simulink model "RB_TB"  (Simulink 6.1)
settings: Solver=ode3  SolverMode=SingleTasking  StartTime=0  StopTime=0.1  FixedStep=0.01  RelTol=1e-3
libraries: simulink x2
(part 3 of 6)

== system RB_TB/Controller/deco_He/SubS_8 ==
  note: Model: RB_TB/Controller/deco_He/SubS_2
  Palv : Inport  Port=1  LatchInput=off
  Pamb_sea : Inport  Port=2  LatchInput=off
  Palv_INI : Inport  Port=3  LatchInput=off
  HT : Inport  Port=4  LatchInput=off
  BC1 : BusCreator  DialogController=Simulink.DDGSource_Bus
  He_a : Constant  Value=0.6508
  He_b : Constant  Value=0.8553
  Mux6 : Mux  Inputs=3
  Product1 : Product
  Sum2 : Sum  Inputs=|+-
  Sum3 : Sum  Inputs=++|
  fcn1 : Fcn  Expr=log(2)/u(1)
  fcn3 : Fcn  Expr=u(3)+u(2)/u(1)
  pr_PHe : TransferFcn  Numerator=[1/60]  Denominator=[1 0]
  bus : Outport
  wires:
  HT/1 -> fcn1/1
  Sum2/1 -> Product1/2
  Product1/1 -> pr_PHe/1
  fcn3/1 -> BC1/4  "M0"
  He_b/1 -> BC1/3, Mux6/1  "He_b"
  Mux6/1 -> fcn3/1
  fcn1/1 -> BC1/1, Product1/1  "He_k"
  Palv/1 -> Sum2/1
  Pamb_sea/1 -> Mux6/2
  He_a/1 -> Mux6/3  "He_a"
  Sum3/1 -> Sum2/2, BC1/2  "Pt"
  Palv_INI/1 -> Sum3/1
  pr_PHe/1 -> Sum3/2
  BC1/1 -> bus/1

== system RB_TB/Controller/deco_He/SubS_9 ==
  note: Model: RB_TB/Controller/deco_He/SubS_2
  Palv : Inport  Port=1  LatchInput=off
  Pamb_sea : Inport  Port=2  LatchInput=off
  Palv_INI : Inport  Port=3  LatchInput=off
  HT : Inport  Port=4  LatchInput=off
  BC1 : BusCreator  DialogController=Simulink.DDGSource_Bus
  He_a : Constant  Value=0.5981
  He_b : Constant  Value=0.8757
  Mux6 : Mux  Inputs=3
  Product1 : Product
  Sum2 : Sum  Inputs=|+-
  Sum3 : Sum  Inputs=++|
  fcn1 : Fcn  Expr=log(2)/u(1)
  fcn3 : Fcn  Expr=u(3)+u(2)/u(1)
  pr_PHe : TransferFcn  Numerator=[1/60]  Denominator=[1 0]
  bus : Outport
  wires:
  BC1/1 -> bus/1
  pr_PHe/1 -> Sum3/2
  Palv_INI/1 -> Sum3/1
  Sum3/1 -> BC1/2, Sum2/2  "Pt"
  He_a/1 -> Mux6/3  "He_a"
  Pamb_sea/1 -> Mux6/2
  Palv/1 -> Sum2/1
  fcn1/1 -> Product1/1, BC1/1  "He_k"
  Mux6/1 -> fcn3/1
  He_b/1 -> Mux6/1, BC1/3  "He_b"
  fcn3/1 -> BC1/4  "M0"
  Product1/1 -> pr_PHe/1
  Sum2/1 -> Product1/2
  HT/1 -> fcn1/1

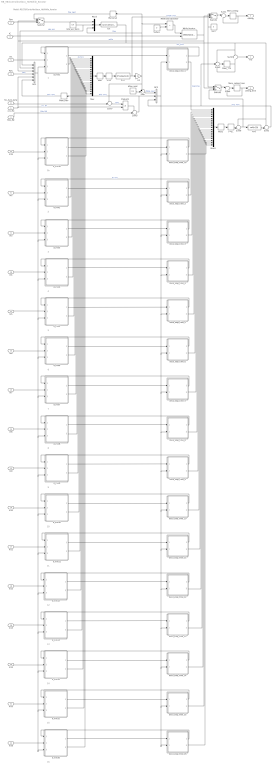
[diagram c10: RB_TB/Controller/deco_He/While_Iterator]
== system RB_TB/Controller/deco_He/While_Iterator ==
  note: 16
  note: 15
  note: 14
  note: 13
  note: 12
  note: 11
  note: 10
  note: 9
  note: 8
  note: 7
  note: 6
  note: 5
  note: 4
  note: 3
  note: 2
  note: 1
  note: Model: RB_TB/Controller/deco_He/While_Iterator
  note: 1b
  cnc_He : Inport  Port=1  LatchInput=off
  Psw : Inport  Port=2  LatchInput=off
  IC : Inport  Port=3  LatchInput=off
  Palv : Inport  Port=4  LatchInput=off
  In1 : Inport  Port=5  LatchInput=off
  In2 : Inport  Port=6  LatchInput=off
  Palv_INI : Inport  Port=7  LatchInput=off
  fnc_hum_temp : Inport  Port=8  LatchInput=off
  In3 : Inport  Port=9  LatchInput=off
  In4 : Inport  Port=10  LatchInput=off
  In5 : Inport  Port=11  LatchInput=off
  In6 : Inport  Port=12  LatchInput=off
  In7 : Inport  Port=13  LatchInput=off
  In8 : Inport  Port=14  LatchInput=off
  In9 : Inport  Port=15  LatchInput=off
  In10 : Inport  Port=16  LatchInput=off
  In11 : Inport  Port=17  LatchInput=off
  In12 : Inport  Port=18  LatchInput=off
  In13 : Inport  Port=19  LatchInput=off
  In14 : Inport  Port=20  LatchInput=off
  In15 : Inport  Port=21  LatchInput=off
  In16 : Inport  Port=22  LatchInput=off
  In1b : Inport  Port=23  LatchInput=off
  >=0 : DeadZone  LowerValue=-1000  UpperValue=0
  >=0_ : DeadZone  LowerValue=-inf  UpperValue=0
  BC1 : BusCreator  DialogController=Simulink.DDGSource_Bus  Inputs=6
  BC2 : BusCreator  DialogController=Simulink.DDGSource_Bus  Inputs=3
  K1 : Gain  Gain=0.1
  Max : MinMax  Function=max
  Max1 : MinMax  Function=max
  Mem_Palv : Memory  Orientation=left  InheritSampleTime=on
  Mem_TTS : Memory  InheritSampleTime=on
  Mem_ceiling : Memory  InheritSampleTime=on
  Mem_ceiling_time : Memory  InheritSampleTime=on
  Memory2 : Memory  Orientation=left  InheritSampleTime=on
  Mux : Mux  Inputs=17
  Mux1 : Mux  Inputs=17
  Mux3 : Mux  Inputs=3
  Product1 : Product
  Relational Operator : RelationalOperator  Operator=>  LogicOutDataTypeMode=Boolean
  Suface : Constant  Value=0
  Sum : Sum  Inputs=+-|
  Sum1 : Sum  Inputs=|++
  Sum2 : Sum  Inputs=-+|
  Sum3 : Sum  Inputs=+++
  Sum4 : Sum  Inputs=|++
  Sum5 : Sum
  Sum6 : Sum  Inputs=++|
  Sum7 : Sum  Inputs=++|
  Sum8 : Sum
  Switch1 : Switch  Threshold=2
  Switch2 : Switch  Threshold=2
  Switch3 : Switch  Threshold=2
  While Iterator : WhileIterator  MaxIters=100  ShowIterationPort=on
  dPsw_next : Constant  Value=0.3
  d_min1 : Subsystem
  d_min10 : Subsystem
  d_min11 : Subsystem
  d_min12 : Subsystem
  d_min13 : Subsystem
  d_min14 : Subsystem
  d_min15 : Subsystem
  d_min16 : Subsystem
  d_min1b : Subsystem
  d_min2 : Subsystem
  d_min3 : Subsystem
  d_min4 : Subsystem
  d_min5 : Subsystem
  d_min6 : Subsystem
  d_min7 : Subsystem
  d_min8 : Subsystem
  d_min9 : Subsystem
  deco_stop_time_1 : Subsystem
  deco_stop_time_10 : Subsystem
  deco_stop_time_11 : Subsystem
  deco_stop_time_12 : Subsystem
  deco_stop_time_13 : Subsystem
  deco_stop_time_14 : Subsystem
  deco_stop_time_15 : Subsystem
  deco_stop_time_16 : Subsystem
  deco_stop_time_1b : Subsystem
  deco_stop_time_2 : Subsystem
  deco_stop_time_3 : Subsystem
  deco_stop_time_4 : Subsystem
  deco_stop_time_5 : Subsystem
  deco_stop_time_6 : Subsystem
  deco_stop_time_7 : Subsystem
  deco_stop_time_8 : Subsystem
  deco_stop_time_9 : Subsystem
  fcn : Fcn  Expr=(u(1)-u(3))/u(2)
  fcn1 : Fcn  Expr=ceil(u(1))
  fcn2 : Fcn  Expr=3*ceil(u(1)/3)
  rate_asc_deco : Constant  Value=0.9
  zero : Constant  Orientation=left  Value=0
  TTS : Outport
  ceiling : Outport  Port=2
  ceiling_time : Outport  Port=3
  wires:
  deco_stop_time_16/2(deco_stop_time) -> Mux1/16
  deco_stop_time_15/2(deco_stop_time) -> Mux1/15
  deco_stop_time_14/2(deco_stop_time) -> Mux1/14
  deco_stop_time_13/2(deco_stop_time) -> Mux1/13
  deco_stop_time_12/2(deco_stop_time) -> Mux1/12
  deco_stop_time_11/2(deco_stop_time) -> Mux1/11
  deco_stop_time_10/2(deco_stop_time) -> Mux1/10
  deco_stop_time_9/2(deco_stop_time) -> Mux1/9
  deco_stop_time_8/2(deco_stop_time) -> Mux1/8
  deco_stop_time_7/2(deco_stop_time) -> Mux1/7
  deco_stop_time_6/2(deco_stop_time) -> Mux1/6
  deco_stop_time_5/2(deco_stop_time) -> Mux1/5
  deco_stop_time_4/2(deco_stop_time) -> Mux1/4
  deco_stop_time_3/2(deco_stop_time) -> Mux1/3
  d_min16/2(d_min) -> Mux/16
  d_min15/2(d_min) -> Mux/15
  d_min14/2(d_min) -> Mux/14
  d_min13/2(d_min) -> Mux/13
  d_min12/2(d_min) -> Mux/12
  d_min11/2(d_min) -> Mux/11
  d_min10/2(d_min) -> Mux/10
  d_min9/2(d_min) -> Mux/9
  d_min8/2(d_min) -> Mux/8
  d_min7/2(d_min) -> Mux/7
  d_min6/2(d_min) -> Mux/6
  d_min5/2(d_min) -> Mux/5
  d_min4/2(d_min) -> Mux/4
  d_min3/2(d_min) -> Mux/3
  deco_stop_time_2/2(deco_stop_time) -> Mux1/2
  Mux1/1 -> Max1/1
  d_min16/1(bus1) -> deco_stop_time_16/1(In1)
  deco_stop_time_16/1(Pt_new) -> d_min16/1(Pt_new)
  In16/1 -> d_min16/2(In1)
  In15/1 -> d_min15/2(In1)
  deco_stop_time_15/1(Pt_new) -> d_min15/1(Pt_new)
  d_min15/1(bus1) -> deco_stop_time_15/1(In1)
  d_min14/1(bus1) -> deco_stop_time_14/1(In1)
  deco_stop_time_14/1(Pt_new) -> d_min14/1(Pt_new)
  In14/1 -> d_min14/2(In1)
  In13/1 -> d_min13/2(In1)
  deco_stop_time_13/1(Pt_new) -> d_min13/1(Pt_new)
  d_min13/1(bus1) -> deco_stop_time_13/1(In1)
  d_min12/1(bus1) -> deco_stop_time_12/1(In1)
  deco_stop_time_12/1(Pt_new) -> d_min12/1(Pt_new)
  In12/1 -> d_min12/2(In1)
  In11/1 -> d_min11/2(In1)
  deco_stop_time_11/1(Pt_new) -> d_min11/1(Pt_new)
  d_min11/1(bus1) -> deco_stop_time_11/1(In1)
  d_min10/1(bus1) -> deco_stop_time_10/1(In1)
  deco_stop_time_10/1(Pt_new) -> d_min10/1(Pt_new)
  In10/1 -> d_min10/2(In1)
  In9/1 -> d_min9/2(In1)
  deco_stop_time_9/1(Pt_new) -> d_min9/1(Pt_new)
  d_min9/1(bus1) -> deco_stop_time_9/1(In1)
  d_min8/1(bus1) -> deco_stop_time_8/1(In1)
  deco_stop_time_8/1(Pt_new) -> d_min8/1(Pt_new)
  In8/1 -> d_min8/2(In1)
  In7/1 -> d_min7/2(In1)
  deco_stop_time_7/1(Pt_new) -> d_min7/1(Pt_new)
  d_min7/1(bus1) -> deco_stop_time_7/1(In1)
  d_min6/1(bus1) -> deco_stop_time_6/1(In1)
  deco_stop_time_6/1(Pt_new) -> d_min6/1(Pt_new)
  In6/1 -> d_min6/2(In1)
  In5/1 -> d_min5/2(In1)
  deco_stop_time_5/1(Pt_new) -> d_min5/1(Pt_new)
  d_min5/1(bus1) -> deco_stop_time_5/1(In1)
  d_min4/1(bus1) -> deco_stop_time_4/1(In1)
  deco_stop_time_4/1(Pt_new) -> d_min4/1(Pt_new)
  In4/1 -> d_min4/2(In1)
  In3/1 -> d_min3/2(In1)
  deco_stop_time_3/1(Pt_new) -> d_min3/1(Pt_new)
  d_min3/1(bus1) -> deco_stop_time_3/1(In1)
  While Iterator/1 -> Switch1/2, Switch3/2, Switch2/2, BC1/3  "while"
  zero/1 -> Switch3/1, Switch1/1
  BC2/1 -> deco_stop_time_1/2(In2), deco_stop_time_16/2(In2), deco_stop_time_15/2(In2), deco_stop_time_14/2(In2), deco_stop_time_13/2(In2), deco_stop_time_12/2(In2), deco_stop_time_11/2(In2), deco_stop_time_10/2(In2), deco_stop_time_9/2(In2), deco_stop_time_8/2(In2), deco_stop_time_7/2(In2), deco_stop_time_6/2(In2), deco_stop_time_5/2(In2), deco_stop_time_4/2(In2), deco_stop_time_3/2(In2), deco_stop_time_2/2(In2), deco_stop_time_1b/2(In2)
  In2/1 -> d_min2/2(In1)
  BC1/1 -> d_min1/3(In2), d_min15/3(In2), d_min16/3(In2), d_min14/3(In2), d_min13/3(In2), d_min12/3(In2), d_min11/3(In2), d_min10/3(In2), d_min9/3(In2), d_min8/3(In2), d_min7/3(In2), d_min6/3(In2), d_min5/3(In2), d_min4/3(In2), d_min3/3(In2), d_min2/3(In2), d_min1b/3(In2)
  Palv/1 -> BC1/4  "Palv"
  Sum8/1 -> TTS/1
  Switch3/1 -> Sum4/1
  Mem_ceiling_time/1 -> ceiling_time/1, Sum4/2
  Sum4/1 -> Mem_ceiling_time/1
  Switch1/1 -> Sum1/1
  Mem_ceiling/1 -> ceiling/1, Sum1/2
  Sum1/1 -> Mem_ceiling/1
  Relational Operator/1 -> While Iterator/1
  Suface/1 -> Relational Operator/2
  >=0_/1 -> Sum6/2
  Sum6/1 -> fcn1/1, Switch3/3
  fcn1/1 -> Sum2/2
  Sum2/1 -> BC2/3, Sum3/2  "stop_time"
  deco_stop_time_2/1(Pt_new) -> d_min2/1(Pt_new)  "Pt_new"
  Sum/1 -> BC2/1  "Pstop_next"
  dPsw_next/1 -> Sum/2
  deco_stop_time_1/1(Pt_new) -> d_min1/1(Pt_new)
  Memory2/1 -> Switch2/1  "Psw_nwxt"
  Switch2/1 -> Mux3/1
  Psw/1 -> Switch2/3
  Mem_Palv/1 -> BC1/6  "Palv_next"
  In1/1 -> d_min1/2(In1)
  d_min2/2(d_min) -> Mux/2
  d_min2/1(bus1) -> deco_stop_time_2/1(In1)
  d_min1/1(bus1) -> deco_stop_time_1/1(In1)
  Sum7/1 -> Product1/1  "Psw'"
  Sum5/1 -> BC2/2, Mem_Palv/1  "Palv_next"
  fnc_hum_temp/1 -> Sum7/2
  Palv_INI/1 -> Sum5/2  "Palv_INI"
  Product1/1 -> Sum5/1
  cnc_He/1 -> BC1/5, Product1/2  "cnc_He"
  Sum3/1 -> Mem_TTS/1
  Mem_TTS/1 -> Sum8/2, Sum3/3
  d_min1/2(d_min) -> Mux/1  "d_min_i"
  fcn/1 -> BC1/1, Sum3/1, Sum8/1, Sum6/1, Sum2/1  "asc_time"
  deco_stop_time_1/2(deco_stop_time) -> Mux1/1  "stop_time_i"
  Mux3/1 -> fcn/1
  Max1/1 -> >=0_/1
  K1/1 -> Relational Operator/1, Memory2/1, Mux3/3, Sum/1, Sum7/1  "Psw"
  rate_asc_deco/1 -> BC1/2, Mux3/2  "rate_asc"
  >=0/1 -> fcn2/1
  Max/1 -> >=0/1
  fcn2/1 -> Switch1/3, K1/1  "Depth_stop"
  IC/1 -> While Iterator/2
  In1b/1 -> d_min1b/2(In1)
  deco_stop_time_1b/1(Pt_new) -> d_min1b/1(Pt_new)
  d_min1b/1(bus1) -> deco_stop_time_1b/1(In1)
  d_min1b/2(d_min) -> Mux/17
  deco_stop_time_1b/2(deco_stop_time) -> Mux1/17
  Mux/1 -> Max/1

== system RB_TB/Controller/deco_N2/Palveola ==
  note: process of Oxygen consumption
  note: RQ = 0.8; 0.9; or 1
  note: Model: RB_TB/Controller/deco_N2/Palveola
  Gas concentration : Inport  Port=1  LatchInput=off
  "depth, m " : Inport  Port=2  LatchInput=off
  RQ : Inport  Port=3  LatchInput=off
  Humidity : Inport  Port=4  LatchInput=off
  Temperature : Inport  Port=5  LatchInput=off
  P_amb_see_level : Inport  Port=6  LatchInput=off
  Fcn : Fcn  Expr=0.0627
  Fcn1 : Fcn  Expr=(1-u(1))/u(1)
  Fcn2 : Fcn  Expr=0
  Mux1 : Mux  Inputs=2
  Product1 : Product
  Product2 : Product
  Product3 : Product
  Sum1 : Sum  Inputs=|+-
  Sum2 : Sum  Inputs=++|
  Sum4 : Sum  Inputs=|++
  Sum5 : Sum  Inputs=++|
  Temperature_see_level : Constant  Value=37
  cnc_N2_atm : Constant  Value=0.78084
  gain1 : Gain  Gain=0.1
  pressure of the CO2 in the lungs  is arterial partial pressure : Constant  Value=0.0534
  Psw : Outport
  Palv : Outport  Port=2
  P_alv_INI : Outport  Port=3
  fnc_hum_temp : Outport  Port=4
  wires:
  "depth, m "/1 -> gain1/1
  Product1/1 -> Sum2/1
  Sum1/1 -> Sum4/1
  Temperature_see_level/1 -> Fcn/1
  pressure of the CO2 in the lungs  is arterial partial pressure/1 -> Product2/2
  Gas concentration/1 -> Product1/1
  RQ/1 -> Fcn1/1
  Fcn1/1 -> Product2/1
  P_amb_see_level/1 -> Sum1/1
  Fcn/1 -> Sum1/2  "Vapor pressure: 0.0627 bar (47 mm Hg)  at 37 degrees Celsius"
  Product2/1 -> Sum4/2
  gain1/1 -> Sum5/1, Psw/1  "pressure of sea water"
  Mux1/1 -> Fcn2/1
  Humidity/1 -> Mux1/1
  Temperature/1 -> Mux1/2
  Sum4/1 -> Product3/2
  cnc_N2_atm/1 -> Product3/1, [cnc_N2_atm]
  Product3/1 -> Sum2/2, P_alv_INI/1  "P_alv_INI"
  Fcn2/1 -> Sum5/2, fnc_hum_temp/1  "fnc_hum_temp"
  Sum5/1 -> Product1/2
  Sum2/1 -> Palv/1  "Alveolar partial pressure of  the gas in the breathing mix"

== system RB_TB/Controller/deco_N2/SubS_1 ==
  note: Pt of seconds
  note: Model: RB_TB/Controller/deco_N2/SubS_X
  Palv : Inport  Port=1  LatchInput=off
  Pamb_sea : Inport  Port=2  LatchInput=off
  Palv_INI : Inport  Port=3  LatchInput=off
  HT : Inport  Port=4  LatchInput=off
  BC1 : BusCreator  DialogController=Simulink.DDGSource_Bus
  Mux6 : Mux  Inputs=3
  Product1 : Product
  Sum2 : Sum  Inputs=|+-
  Sum3 : Sum  Inputs=++|
  fcn3 : Fcn  Expr=u(3)+u(2)/u(1)
  fcn5 : Fcn  Expr=log(2)/u(1)
  fcn6 : Fcn  Expr=1.005-u(1)^(-1/2)
  fcn7 : Fcn  Expr=2*u(1)^(-1/3)
  pr_PN2 : TransferFcn  Numerator=[1/60]  Denominator=[1 0]
  bus : Outport
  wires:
  Sum2/1 -> Product1/2
  Product1/1 -> pr_PN2/1
  fcn3/1 -> BC1/4  "M0"
  fcn6/1 -> Mux6/1, BC1/3  "N2_b"
  Mux6/1 -> fcn3/1
  fcn5/1 -> Product1/1, BC1/1  "N2_k"
  Palv/1 -> Sum2/1
  Pamb_sea/1 -> Mux6/2
  fcn7/1 -> Mux6/3  "N2_a"
  Sum3/1 -> BC1/2, Sum2/2  "Pt"
  Palv_INI/1 -> Sum3/1
  pr_PN2/1 -> Sum3/2
  BC1/1 -> bus/1
  HT/1 -> fcn7/1, fcn5/1, fcn6/1

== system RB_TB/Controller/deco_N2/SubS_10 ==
  note: Model: RB_TB/Controller/deco_N2/SubS_X
  note: Pt of seconds
  Palv : Inport  Port=1  LatchInput=off
  Pamb_sea : Inport  Port=2  LatchInput=off
  Palv_INI : Inport  Port=3  LatchInput=off
  HT : Inport  Port=4  LatchInput=off
  BC1 : BusCreator  DialogController=Simulink.DDGSource_Bus
  Mux6 : Mux  Inputs=3
  Product1 : Product
  Sum2 : Sum  Inputs=|+-
  Sum3 : Sum  Inputs=++|
  fcn3 : Fcn  Expr=u(3)+u(2)/u(1)
  fcn5 : Fcn  Expr=log(2)/u(1)
  fcn6 : Fcn  Expr=1.005-u(1)^(-1/2)
  fcn7 : Fcn  Expr=2*u(1)^(-1/3)
  pr_PN2 : TransferFcn  Numerator=[1/60]  Denominator=[1 0]
  bus : Outport
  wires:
  HT/1 -> fcn6/1, fcn5/1, fcn7/1
  BC1/1 -> bus/1
  pr_PN2/1 -> Sum3/2
  Palv_INI/1 -> Sum3/1
  Sum3/1 -> Sum2/2, BC1/2  "Pt"
  fcn7/1 -> Mux6/3  "N2_a"
  Pamb_sea/1 -> Mux6/2
  Palv/1 -> Sum2/1
  fcn5/1 -> BC1/1, Product1/1  "N2_k"
  Mux6/1 -> fcn3/1
  fcn6/1 -> BC1/3, Mux6/1  "N2_b"
  fcn3/1 -> BC1/4  "M0"
  Product1/1 -> pr_PN2/1
  Sum2/1 -> Product1/2

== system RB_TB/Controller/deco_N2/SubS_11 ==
  note: Pt of seconds
  note: Model: RB_TB/Controller/deco_N2/SubS_X
  Palv : Inport  Port=1  LatchInput=off
  Pamb_sea : Inport  Port=2  LatchInput=off
  Palv_INI : Inport  Port=3  LatchInput=off
  HT : Inport  Port=4  LatchInput=off
  BC1 : BusCreator  DialogController=Simulink.DDGSource_Bus
  Mux6 : Mux  Inputs=3
  Product1 : Product
  Sum2 : Sum  Inputs=|+-
  Sum3 : Sum  Inputs=++|
  fcn3 : Fcn  Expr=u(3)+u(2)/u(1)
  fcn5 : Fcn  Expr=log(2)/u(1)
  fcn6 : Fcn  Expr=1.005-u(1)^(-1/2)
  fcn7 : Fcn  Expr=2*u(1)^(-1/3)
  pr_PN2 : TransferFcn  Numerator=[1/60]  Denominator=[1 0]
  bus : Outport
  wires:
  Sum2/1 -> Product1/2
  Product1/1 -> pr_PN2/1
  fcn3/1 -> BC1/4  "M0"
  fcn6/1 -> Mux6/1, BC1/3  "N2_b"
  Mux6/1 -> fcn3/1
  fcn5/1 -> Product1/1, BC1/1  "N2_k"
  Palv/1 -> Sum2/1
  Pamb_sea/1 -> Mux6/2
  fcn7/1 -> Mux6/3  "N2_a"
  Sum3/1 -> BC1/2, Sum2/2  "Pt"
  Palv_INI/1 -> Sum3/1
  pr_PN2/1 -> Sum3/2
  BC1/1 -> bus/1
  HT/1 -> fcn7/1, fcn5/1, fcn6/1

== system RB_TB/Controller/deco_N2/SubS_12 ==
  note: Model: RB_TB/Controller/deco_N2/SubS_X
  note: Pt of seconds
  Palv : Inport  Port=1  LatchInput=off
  Pamb_sea : Inport  Port=2  LatchInput=off
  Palv_INI : Inport  Port=3  LatchInput=off
  HT : Inport  Port=4  LatchInput=off
  BC1 : BusCreator  DialogController=Simulink.DDGSource_Bus
  Mux6 : Mux  Inputs=3
  Product1 : Product
  Sum2 : Sum  Inputs=|+-
  Sum3 : Sum  Inputs=++|
  fcn3 : Fcn  Expr=u(3)+u(2)/u(1)
  fcn5 : Fcn  Expr=log(2)/u(1)
  fcn6 : Fcn  Expr=1.005-u(1)^(-1/2)
  fcn7 : Fcn  Expr=2*u(1)^(-1/3)
  pr_PN2 : TransferFcn  Numerator=[1/60]  Denominator=[1 0]
  bus : Outport
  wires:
  HT/1 -> fcn6/1, fcn5/1, fcn7/1
  BC1/1 -> bus/1
  pr_PN2/1 -> Sum3/2
  Palv_INI/1 -> Sum3/1
  Sum3/1 -> Sum2/2, BC1/2  "Pt"
  fcn7/1 -> Mux6/3  "N2_a"
  Pamb_sea/1 -> Mux6/2
  Palv/1 -> Sum2/1
  fcn5/1 -> BC1/1, Product1/1  "N2_k"
  Mux6/1 -> fcn3/1
  fcn6/1 -> BC1/3, Mux6/1  "N2_b"
  fcn3/1 -> BC1/4  "M0"
  Product1/1 -> pr_PN2/1
  Sum2/1 -> Product1/2

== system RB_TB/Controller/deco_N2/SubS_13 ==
  note: Pt of seconds
  note: Model: RB_TB/Controller/deco_N2/SubS_X
  Palv : Inport  Port=1  LatchInput=off
  Pamb_sea : Inport  Port=2  LatchInput=off
  Palv_INI : Inport  Port=3  LatchInput=off
  HT : Inport  Port=4  LatchInput=off
  BC1 : BusCreator  DialogController=Simulink.DDGSource_Bus
  Mux6 : Mux  Inputs=3
  Product1 : Product
  Sum2 : Sum  Inputs=|+-
  Sum3 : Sum  Inputs=++|
  fcn3 : Fcn  Expr=u(3)+u(2)/u(1)
  fcn5 : Fcn  Expr=log(2)/u(1)
  fcn6 : Fcn  Expr=1.005-u(1)^(-1/2)
  fcn7 : Fcn  Expr=2*u(1)^(-1/3)
  pr_PN2 : TransferFcn  Numerator=[1/60]  Denominator=[1 0]
  bus : Outport
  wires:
  Sum2/1 -> Product1/2
  Product1/1 -> pr_PN2/1
  fcn3/1 -> BC1/4  "M0"
  fcn6/1 -> Mux6/1, BC1/3  "N2_b"
  Mux6/1 -> fcn3/1
  fcn5/1 -> Product1/1, BC1/1  "N2_k"
  Palv/1 -> Sum2/1
  Pamb_sea/1 -> Mux6/2
  fcn7/1 -> Mux6/3  "N2_a"
  Sum3/1 -> BC1/2, Sum2/2  "Pt"
  Palv_INI/1 -> Sum3/1
  pr_PN2/1 -> Sum3/2
  BC1/1 -> bus/1
  HT/1 -> fcn7/1, fcn5/1, fcn6/1

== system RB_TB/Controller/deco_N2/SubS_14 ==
  note: Model: RB_TB/Controller/deco_N2/SubS_X
  note: Pt of seconds
  Palv : Inport  Port=1  LatchInput=off
  Pamb_sea : Inport  Port=2  LatchInput=off
  Palv_INI : Inport  Port=3  LatchInput=off
  HT : Inport  Port=4  LatchInput=off
  BC1 : BusCreator  DialogController=Simulink.DDGSource_Bus
  Mux6 : Mux  Inputs=3
  Product1 : Product
  Sum2 : Sum  Inputs=|+-
  Sum3 : Sum  Inputs=++|
  fcn3 : Fcn  Expr=u(3)+u(2)/u(1)
  fcn5 : Fcn  Expr=log(2)/u(1)
  fcn6 : Fcn  Expr=1.005-u(1)^(-1/2)
  fcn7 : Fcn  Expr=2*u(1)^(-1/3)
  pr_PN2 : TransferFcn  Numerator=[1/60]  Denominator=[1 0]
  bus : Outport
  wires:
  HT/1 -> fcn6/1, fcn5/1, fcn7/1
  BC1/1 -> bus/1
  pr_PN2/1 -> Sum3/2
  Palv_INI/1 -> Sum3/1
  Sum3/1 -> Sum2/2, BC1/2  "Pt"
  fcn7/1 -> Mux6/3  "N2_a"
  Pamb_sea/1 -> Mux6/2
  Palv/1 -> Sum2/1
  fcn5/1 -> BC1/1, Product1/1  "N2_k"
  Mux6/1 -> fcn3/1
  fcn6/1 -> BC1/3, Mux6/1  "N2_b"
  fcn3/1 -> BC1/4  "M0"
  Product1/1 -> pr_PN2/1
  Sum2/1 -> Product1/2

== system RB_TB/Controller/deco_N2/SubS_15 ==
  note: Pt of seconds
  note: Model: RB_TB/Controller/deco_N2/SubS_X
  Palv : Inport  Port=1  LatchInput=off
  Pamb_sea : Inport  Port=2  LatchInput=off
  Palv_INI : Inport  Port=3  LatchInput=off
  HT : Inport  Port=4  LatchInput=off
  BC1 : BusCreator  DialogController=Simulink.DDGSource_Bus
  Mux6 : Mux  Inputs=3
  Product1 : Product
  Sum2 : Sum  Inputs=|+-
  Sum3 : Sum  Inputs=++|
  fcn3 : Fcn  Expr=u(3)+u(2)/u(1)
  fcn5 : Fcn  Expr=log(2)/u(1)
  fcn6 : Fcn  Expr=1.005-u(1)^(-1/2)
  fcn7 : Fcn  Expr=2*u(1)^(-1/3)
  pr_PN2 : TransferFcn  Numerator=[1/60]  Denominator=[1 0]
  bus : Outport
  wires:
  Sum2/1 -> Product1/2
  Product1/1 -> pr_PN2/1
  fcn3/1 -> BC1/4  "M0"
  fcn6/1 -> Mux6/1, BC1/3  "N2_b"
  Mux6/1 -> fcn3/1
  fcn5/1 -> Product1/1, BC1/1  "N2_k"
  Palv/1 -> Sum2/1
  Pamb_sea/1 -> Mux6/2
  fcn7/1 -> Mux6/3  "N2_a"
  Sum3/1 -> BC1/2, Sum2/2  "Pt"
  Palv_INI/1 -> Sum3/1
  pr_PN2/1 -> Sum3/2
  BC1/1 -> bus/1
  HT/1 -> fcn7/1, fcn5/1, fcn6/1

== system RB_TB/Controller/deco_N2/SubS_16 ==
  note: Model: RB_TB/Controller/deco_N2/SubS_X
  note: Pt of seconds
  Palv : Inport  Port=1  LatchInput=off
  Pamb_sea : Inport  Port=2  LatchInput=off
  Palv_INI : Inport  Port=3  LatchInput=off
  HT : Inport  Port=4  LatchInput=off
  BC1 : BusCreator  DialogController=Simulink.DDGSource_Bus
  Mux6 : Mux  Inputs=3
  Product1 : Product
  Sum2 : Sum  Inputs=|+-
  Sum3 : Sum  Inputs=++|
  fcn3 : Fcn  Expr=u(3)+u(2)/u(1)
  fcn5 : Fcn  Expr=log(2)/u(1)
  fcn6 : Fcn  Expr=1.005-u(1)^(-1/2)
  fcn7 : Fcn  Expr=2*u(1)^(-1/3)
  pr_PN2 : TransferFcn  Numerator=[1/60]  Denominator=[1 0]
  bus : Outport
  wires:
  HT/1 -> fcn6/1, fcn5/1, fcn7/1
  BC1/1 -> bus/1
  pr_PN2/1 -> Sum3/2
  Palv_INI/1 -> Sum3/1
  Sum3/1 -> Sum2/2, BC1/2  "Pt"
  fcn7/1 -> Mux6/3  "N2_a"
  Pamb_sea/1 -> Mux6/2
  Palv/1 -> Sum2/1
  fcn5/1 -> BC1/1, Product1/1  "N2_k"
  Mux6/1 -> fcn3/1
  fcn6/1 -> BC1/3, Mux6/1  "N2_b"
  fcn3/1 -> BC1/4  "M0"
  Product1/1 -> pr_PN2/1
  Sum2/1 -> Product1/2

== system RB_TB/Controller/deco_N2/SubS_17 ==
  note: Pt of seconds
  note: Model: RB_TB/Controller/deco_N2/SubS_X
  Palv : Inport  Port=1  LatchInput=off
  Pamb_sea : Inport  Port=2  LatchInput=off
  Palv_INI : Inport  Port=3  LatchInput=off
  HT : Inport  Port=4  LatchInput=off
  BC1 : BusCreator  DialogController=Simulink.DDGSource_Bus
  Mux6 : Mux  Inputs=3
  Product1 : Product
  Sum2 : Sum  Inputs=|+-
  Sum3 : Sum  Inputs=++|
  fcn3 : Fcn  Expr=u(3)+u(2)/u(1)
  fcn5 : Fcn  Expr=log(2)/u(1)
  fcn6 : Fcn  Expr=1.005-u(1)^(-1/2)
  fcn7 : Fcn  Expr=2*u(1)^(-1/3)
  pr_PN2 : TransferFcn  Numerator=[1/60]  Denominator=[1 0]
  bus : Outport
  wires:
  Sum2/1 -> Product1/2
  Product1/1 -> pr_PN2/1
  fcn3/1 -> BC1/4  "M0"
  fcn6/1 -> Mux6/1, BC1/3  "N2_b"
  Mux6/1 -> fcn3/1
  fcn5/1 -> Product1/1, BC1/1  "N2_k"
  Palv/1 -> Sum2/1
  Pamb_sea/1 -> Mux6/2
  fcn7/1 -> Mux6/3  "N2_a"
  Sum3/1 -> BC1/2, Sum2/2  "Pt"
  Palv_INI/1 -> Sum3/1
  pr_PN2/1 -> Sum3/2
  BC1/1 -> bus/1
  HT/1 -> fcn7/1, fcn5/1, fcn6/1

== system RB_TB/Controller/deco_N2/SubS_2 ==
  note: Model: RB_TB/Controller/deco_N2/SubS_X
  note: Pt of seconds
  Palv : Inport  Port=1  LatchInput=off
  Pamb_sea : Inport  Port=2  LatchInput=off
  Palv_INI : Inport  Port=3  LatchInput=off
  HT : Inport  Port=4  LatchInput=off
  BC1 : BusCreator  DialogController=Simulink.DDGSource_Bus
  Mux6 : Mux  Inputs=3
  Product1 : Product
  Sum2 : Sum  Inputs=|+-
  Sum3 : Sum  Inputs=++|
  fcn3 : Fcn  Expr=u(3)+u(2)/u(1)
  fcn5 : Fcn  Expr=log(2)/u(1)
  fcn6 : Fcn  Expr=1.005-u(1)^(-1/2)
  fcn7 : Fcn  Expr=2*u(1)^(-1/3)
  pr_PN2 : TransferFcn  Numerator=[1/60]  Denominator=[1 0]
  bus : Outport
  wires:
  HT/1 -> fcn6/1, fcn5/1, fcn7/1
  BC1/1 -> bus/1
  pr_PN2/1 -> Sum3/2
  Palv_INI/1 -> Sum3/1
  Sum3/1 -> Sum2/2, BC1/2  "Pt"
  fcn7/1 -> Mux6/3  "N2_a"
  Pamb_sea/1 -> Mux6/2
  Palv/1 -> Sum2/1
  fcn5/1 -> BC1/1, Product1/1  "N2_k"
  Mux6/1 -> fcn3/1
  fcn6/1 -> BC1/3, Mux6/1  "N2_b"
  fcn3/1 -> BC1/4  "M0"
  Product1/1 -> pr_PN2/1
  Sum2/1 -> Product1/2

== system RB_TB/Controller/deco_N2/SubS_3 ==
  note: Pt of seconds
  note: Model: RB_TB/Controller/deco_N2/SubS_X
  Palv : Inport  Port=1  LatchInput=off
  Pamb_sea : Inport  Port=2  LatchInput=off
  Palv_INI : Inport  Port=3  LatchInput=off
  HT : Inport  Port=4  LatchInput=off
  BC1 : BusCreator  DialogController=Simulink.DDGSource_Bus
  Mux6 : Mux  Inputs=3
  Product1 : Product
  Sum2 : Sum  Inputs=|+-
  Sum3 : Sum  Inputs=++|
  fcn3 : Fcn  Expr=u(3)+u(2)/u(1)
  fcn5 : Fcn  Expr=log(2)/u(1)
  fcn6 : Fcn  Expr=1.005-u(1)^(-1/2)
  fcn7 : Fcn  Expr=2*u(1)^(-1/3)
  pr_PN2 : TransferFcn  Numerator=[1/60]  Denominator=[1 0]
  bus : Outport
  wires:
  Sum2/1 -> Product1/2
  Product1/1 -> pr_PN2/1
  fcn3/1 -> BC1/4  "M0"
  fcn6/1 -> Mux6/1, BC1/3  "N2_b"
  Mux6/1 -> fcn3/1
  fcn5/1 -> Product1/1, BC1/1  "N2_k"
  Palv/1 -> Sum2/1
  Pamb_sea/1 -> Mux6/2
  fcn7/1 -> Mux6/3  "N2_a"
  Sum3/1 -> BC1/2, Sum2/2  "Pt"
  Palv_INI/1 -> Sum3/1
  pr_PN2/1 -> Sum3/2
  BC1/1 -> bus/1
  HT/1 -> fcn7/1, fcn5/1, fcn6/1

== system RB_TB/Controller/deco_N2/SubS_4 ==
  note: Model: RB_TB/Controller/deco_N2/SubS_X
  note: Pt of seconds
  Palv : Inport  Port=1  LatchInput=off
  Pamb_sea : Inport  Port=2  LatchInput=off
  Palv_INI : Inport  Port=3  LatchInput=off
  HT : Inport  Port=4  LatchInput=off
  BC1 : BusCreator  DialogController=Simulink.DDGSource_Bus
  Mux6 : Mux  Inputs=3
  Product1 : Product
  Sum2 : Sum  Inputs=|+-
  Sum3 : Sum  Inputs=++|
  fcn3 : Fcn  Expr=u(3)+u(2)/u(1)
  fcn5 : Fcn  Expr=log(2)/u(1)
  fcn6 : Fcn  Expr=1.005-u(1)^(-1/2)
  fcn7 : Fcn  Expr=2*u(1)^(-1/3)
  pr_PN2 : TransferFcn  Numerator=[1/60]  Denominator=[1 0]
  bus : Outport
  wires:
  HT/1 -> fcn6/1, fcn5/1, fcn7/1
  BC1/1 -> bus/1
  pr_PN2/1 -> Sum3/2
  Palv_INI/1 -> Sum3/1
  Sum3/1 -> Sum2/2, BC1/2  "Pt"
  fcn7/1 -> Mux6/3  "N2_a"
  Pamb_sea/1 -> Mux6/2
  Palv/1 -> Sum2/1
  fcn5/1 -> BC1/1, Product1/1  "N2_k"
  Mux6/1 -> fcn3/1
  fcn6/1 -> BC1/3, Mux6/1  "N2_b"
  fcn3/1 -> BC1/4  "M0"
  Product1/1 -> pr_PN2/1
  Sum2/1 -> Product1/2

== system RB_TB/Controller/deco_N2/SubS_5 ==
  note: Pt of seconds
  note: Model: RB_TB/Controller/deco_N2/SubS_X
  Palv : Inport  Port=1  LatchInput=off
  Pamb_sea : Inport  Port=2  LatchInput=off
  Palv_INI : Inport  Port=3  LatchInput=off
  HT : Inport  Port=4  LatchInput=off
  BC1 : BusCreator  DialogController=Simulink.DDGSource_Bus
  Mux6 : Mux  Inputs=3
  Product1 : Product
  Sum2 : Sum  Inputs=|+-
  Sum3 : Sum  Inputs=++|
  fcn3 : Fcn  Expr=u(3)+u(2)/u(1)
  fcn5 : Fcn  Expr=log(2)/u(1)
  fcn6 : Fcn  Expr=1.005-u(1)^(-1/2)
  fcn7 : Fcn  Expr=2*u(1)^(-1/3)
  pr_PN2 : TransferFcn  Numerator=[1/60]  Denominator=[1 0]
  bus : Outport
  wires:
  Sum2/1 -> Product1/2
  Product1/1 -> pr_PN2/1
  fcn3/1 -> BC1/4  "M0"
  fcn6/1 -> Mux6/1, BC1/3  "N2_b"
  Mux6/1 -> fcn3/1
  fcn5/1 -> Product1/1, BC1/1  "N2_k"
  Palv/1 -> Sum2/1
  Pamb_sea/1 -> Mux6/2
  fcn7/1 -> Mux6/3  "N2_a"
  Sum3/1 -> BC1/2, Sum2/2  "Pt"
  Palv_INI/1 -> Sum3/1
  pr_PN2/1 -> Sum3/2
  BC1/1 -> bus/1
  HT/1 -> fcn7/1, fcn5/1, fcn6/1

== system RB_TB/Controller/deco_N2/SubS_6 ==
  note: Model: RB_TB/Controller/deco_N2/SubS_X
  note: Pt of seconds
  Palv : Inport  Port=1  LatchInput=off
  Pamb_sea : Inport  Port=2  LatchInput=off
  Palv_INI : Inport  Port=3  LatchInput=off
  HT : Inport  Port=4  LatchInput=off
  BC1 : BusCreator  DialogController=Simulink.DDGSource_Bus
  Mux6 : Mux  Inputs=3
  Product1 : Product
  Sum2 : Sum  Inputs=|+-
  Sum3 : Sum  Inputs=++|
  fcn3 : Fcn  Expr=u(3)+u(2)/u(1)
  fcn5 : Fcn  Expr=log(2)/u(1)
  fcn6 : Fcn  Expr=1.005-u(1)^(-1/2)
  fcn7 : Fcn  Expr=2*u(1)^(-1/3)
  pr_PN2 : TransferFcn  Numerator=[1/60]  Denominator=[1 0]
  bus : Outport
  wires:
  HT/1 -> fcn6/1, fcn5/1, fcn7/1
  BC1/1 -> bus/1
  pr_PN2/1 -> Sum3/2
  Palv_INI/1 -> Sum3/1
  Sum3/1 -> Sum2/2, BC1/2  "Pt"
  fcn7/1 -> Mux6/3  "N2_a"
  Pamb_sea/1 -> Mux6/2
  Palv/1 -> Sum2/1
  fcn5/1 -> BC1/1, Product1/1  "N2_k"
  Mux6/1 -> fcn3/1
  fcn6/1 -> BC1/3, Mux6/1  "N2_b"
  fcn3/1 -> BC1/4  "M0"
  Product1/1 -> pr_PN2/1
  Sum2/1 -> Product1/2

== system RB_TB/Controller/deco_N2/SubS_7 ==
  note: Pt of seconds
  note: Model: RB_TB/Controller/deco_N2/SubS_X
  Palv : Inport  Port=1  LatchInput=off
  Pamb_sea : Inport  Port=2  LatchInput=off
  Palv_INI : Inport  Port=3  LatchInput=off
  HT : Inport  Port=4  LatchInput=off
  BC1 : BusCreator  DialogController=Simulink.DDGSource_Bus
  Mux6 : Mux  Inputs=3
  Product1 : Product
  Sum2 : Sum  Inputs=|+-
  Sum3 : Sum  Inputs=++|
  fcn3 : Fcn  Expr=u(3)+u(2)/u(1)
  fcn5 : Fcn  Expr=log(2)/u(1)
  fcn6 : Fcn  Expr=1.005-u(1)^(-1/2)
  fcn7 : Fcn  Expr=2*u(1)^(-1/3)
  pr_PN2 : TransferFcn  Numerator=[1/60]  Denominator=[1 0]
  bus : Outport
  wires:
  Sum2/1 -> Product1/2
  Product1/1 -> pr_PN2/1
  fcn3/1 -> BC1/4  "M0"
  fcn6/1 -> Mux6/1, BC1/3  "N2_b"
  Mux6/1 -> fcn3/1
  fcn5/1 -> Product1/1, BC1/1  "N2_k"
  Palv/1 -> Sum2/1
  Pamb_sea/1 -> Mux6/2
  fcn7/1 -> Mux6/3  "N2_a"
  Sum3/1 -> BC1/2, Sum2/2  "Pt"
  Palv_INI/1 -> Sum3/1
  pr_PN2/1 -> Sum3/2
  BC1/1 -> bus/1
  HT/1 -> fcn7/1, fcn5/1, fcn6/1

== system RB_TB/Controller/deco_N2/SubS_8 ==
  note: Model: RB_TB/Controller/deco_N2/SubS_X
  note: Pt of seconds
  Palv : Inport  Port=1  LatchInput=off
  Pamb_sea : Inport  Port=2  LatchInput=off
  Palv_INI : Inport  Port=3  LatchInput=off
  HT : Inport  Port=4  LatchInput=off
  BC1 : BusCreator  DialogController=Simulink.DDGSource_Bus
  Mux6 : Mux  Inputs=3
  Product1 : Product
  Sum2 : Sum  Inputs=|+-
  Sum3 : Sum  Inputs=++|
  fcn3 : Fcn  Expr=u(3)+u(2)/u(1)
  fcn5 : Fcn  Expr=log(2)/u(1)
  fcn6 : Fcn  Expr=1.005-u(1)^(-1/2)
  fcn7 : Fcn  Expr=2*u(1)^(-1/3)
  pr_PN2 : TransferFcn  Numerator=[1/60]  Denominator=[1 0]
  bus : Outport
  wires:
  HT/1 -> fcn6/1, fcn5/1, fcn7/1
  BC1/1 -> bus/1
  pr_PN2/1 -> Sum3/2
  Palv_INI/1 -> Sum3/1
  Sum3/1 -> Sum2/2, BC1/2  "Pt"
  fcn7/1 -> Mux6/3  "N2_a"
  Pamb_sea/1 -> Mux6/2
  Palv/1 -> Sum2/1
  fcn5/1 -> BC1/1, Product1/1  "N2_k"
  Mux6/1 -> fcn3/1
  fcn6/1 -> BC1/3, Mux6/1  "N2_b"
  fcn3/1 -> BC1/4  "M0"
  Product1/1 -> pr_PN2/1
  Sum2/1 -> Product1/2

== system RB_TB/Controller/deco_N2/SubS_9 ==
  note: Pt of seconds
  note: Model: RB_TB/Controller/deco_N2/SubS_X
  Palv : Inport  Port=1  LatchInput=off
  Pamb_sea : Inport  Port=2  LatchInput=off
  Palv_INI : Inport  Port=3  LatchInput=off
  HT : Inport  Port=4  LatchInput=off
  BC1 : BusCreator  DialogController=Simulink.DDGSource_Bus
  Mux6 : Mux  Inputs=3
  Product1 : Product
  Sum2 : Sum  Inputs=|+-
  Sum3 : Sum  Inputs=++|
  fcn3 : Fcn  Expr=u(3)+u(2)/u(1)
  fcn5 : Fcn  Expr=log(2)/u(1)
  fcn6 : Fcn  Expr=1.005-u(1)^(-1/2)
  fcn7 : Fcn  Expr=2*u(1)^(-1/3)
  pr_PN2 : TransferFcn  Numerator=[1/60]  Denominator=[1 0]
  bus : Outport
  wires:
  Sum2/1 -> Product1/2
  Product1/1 -> pr_PN2/1
  fcn3/1 -> BC1/4  "M0"
  fcn6/1 -> Mux6/1, BC1/3  "N2_b"
  Mux6/1 -> fcn3/1
  fcn5/1 -> Product1/1, BC1/1  "N2_k"
  Palv/1 -> Sum2/1
  Pamb_sea/1 -> Mux6/2
  fcn7/1 -> Mux6/3  "N2_a"
  Sum3/1 -> BC1/2, Sum2/2  "Pt"
  Palv_INI/1 -> Sum3/1
  pr_PN2/1 -> Sum3/2
  BC1/1 -> bus/1
  HT/1 -> fcn7/1, fcn5/1, fcn6/1

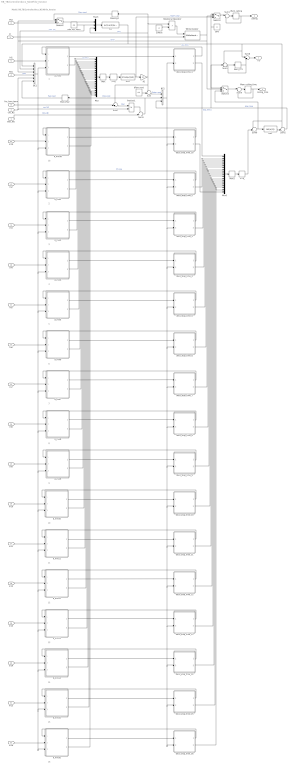
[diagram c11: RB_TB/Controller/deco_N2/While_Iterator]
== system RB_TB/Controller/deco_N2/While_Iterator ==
  note: 1
  note: 2
  note: 3
  note: 4
  note: 5
  note: 6
  note: 7
  note: 8
  note: 9
  note: 10
  note: 11
  note: 12
  note: 13
  note: 14
  note: 15
  note: 16
  note: Model: RB_TB/Controller/deco_N2/While_Iterator
  note: 1b
  cnc_N2 : Inport  Port=1  LatchInput=off
  Psw : Inport  Port=2  LatchInput=off
  IC : Inport  Port=3  LatchInput=off
  Palv : Inport  Port=4  LatchInput=off
  In1 : Inport  Port=5  LatchInput=off
  In2 : Inport  Port=6  LatchInput=off
  Palv_INI : Inport  Port=7  LatchInput=off
  fnc_hum_temp : Inport  Port=8  LatchInput=off
  In3 : Inport  Port=9  LatchInput=off
  In4 : Inport  Port=10  LatchInput=off
  In5 : Inport  Port=11  LatchInput=off
  In6 : Inport  Port=12  LatchInput=off
  In7 : Inport  Port=13  LatchInput=off
  In8 : Inport  Port=14  LatchInput=off
  In9 : Inport  Port=15  LatchInput=off
  In10 : Inport  Port=16  LatchInput=off
  In11 : Inport  Port=17  LatchInput=off
  In12 : Inport  Port=18  LatchInput=off
  In13 : Inport  Port=19  LatchInput=off
  In14 : Inport  Port=20  LatchInput=off
  In15 : Inport  Port=21  LatchInput=off
  In16 : Inport  Port=22  LatchInput=off
  In1b : Inport  Port=23  LatchInput=off
  >=0 : DeadZone  LowerValue=-1000  UpperValue=0
  >=0_ : DeadZone  LowerValue=-inf  UpperValue=0
  BC1 : BusCreator  DialogController=Simulink.DDGSource_Bus  Inputs=6
  BC2 : BusCreator  DialogController=Simulink.DDGSource_Bus  Inputs=3
  K1 : Gain  Gain=0.1
  Max : MinMax  Function=max
  Max1 : MinMax  Function=max
  Mem_Palv : Memory  Orientation=left  InheritSampleTime=on
  Mem_TTS : Memory  InheritSampleTime=on
  Mem_ceiling : Memory  InheritSampleTime=on
  Mem_ceiling_time : Memory  InheritSampleTime=on
  Memory2 : Memory  Orientation=left  InheritSampleTime=on
  Mux : Mux  Inputs=17
  Mux1 : Mux  Inputs=17
  Mux3 : Mux  Inputs=3
  Product1 : Product
  Relational Operator : RelationalOperator  Operator=>  LogicOutDataTypeMode=Boolean
  Suface : Constant  Value=0
  Sum : Sum  Inputs=+-|
  Sum1 : Sum  Inputs=|++
  Sum2 : Sum  Inputs=-+|
  Sum3 : Sum  Inputs=+++
  Sum4 : Sum  Inputs=|++
  Sum5 : Sum
  Sum6 : Sum  Inputs=++|
  Sum7 : Sum  Inputs=++|
  Sum8 : Sum
  Switch1 : Switch  Threshold=2
  Switch2 : Switch  Threshold=2
  Switch3 : Switch  Threshold=2
  While Iterator : WhileIterator  MaxIters=100  ShowIterationPort=on
  dPsw_next : Constant  Value=0.3
  d_min1 : Subsystem
  d_min10 : Subsystem
  d_min11 : Subsystem
  d_min12 : Subsystem
  d_min13 : Subsystem
  d_min14 : Subsystem
  d_min15 : Subsystem
  d_min16 : Subsystem
  d_min1b : Subsystem
  d_min2 : Subsystem
  d_min3 : Subsystem
  d_min4 : Subsystem
  d_min5 : Subsystem
  d_min6 : Subsystem
  d_min7 : Subsystem
  d_min8 : Subsystem
  d_min9 : Subsystem
  deco_stop_time_1 : Subsystem
  deco_stop_time_10 : Subsystem
  deco_stop_time_11 : Subsystem
  deco_stop_time_12 : Subsystem
  deco_stop_time_13 : Subsystem
  deco_stop_time_14 : Subsystem
  deco_stop_time_15 : Subsystem
  deco_stop_time_16 : Subsystem
  deco_stop_time_1b : Subsystem
  deco_stop_time_2 : Subsystem
  deco_stop_time_3 : Subsystem
  deco_stop_time_4 : Subsystem
  deco_stop_time_5 : Subsystem
  deco_stop_time_6 : Subsystem
  deco_stop_time_7 : Subsystem
  deco_stop_time_8 : Subsystem
  deco_stop_time_9 : Subsystem
  fcn : Fcn  Expr=(u(1)-u(3))/u(2)
  fcn1 : Fcn  Expr=ceil(u(1))
  fcn2 : Fcn  Expr=3*ceil(u(1)/3)
  rate_asc_deco : Constant  Value=0.9
  zero : Constant  Orientation=left  Value=0
  TTS : Outport
  ceiling : Outport  Port=2
  ceiling_time : Outport  Port=3
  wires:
  IC/1 -> While Iterator/2
  Mux/1 -> Max/1
  fcn2/1 -> K1/1, Switch1/3  "Depth_stop"
  Max/1 -> >=0/1
  >=0/1 -> fcn2/1
  rate_asc_deco/1 -> Mux3/2, BC1/2  "rate_asc"
  K1/1 -> Sum7/1, Sum/1, Mux3/3, Memory2/1, Relational Operator/1  "Psw"
  Max1/1 -> >=0_/1
  Mux3/1 -> fcn/1
  deco_stop_time_1/2(deco_stop_time) -> Mux1/1  "stop_time_i"
  fcn/1 -> Sum8/1, Sum3/1, Sum2/1, Sum6/1, BC1/1  "asc_time"
  d_min1/2(d_min) -> Mux/1  "d_min_i"
  Mem_TTS/1 -> Sum8/2, Sum3/3
  Sum3/1 -> Mem_TTS/1
  cnc_N2/1 -> Product1/2, BC1/5  "cnc_N2"
  Product1/1 -> Sum5/1
  Palv_INI/1 -> Sum5/2  "Palv_INI"
  fnc_hum_temp/1 -> Sum7/2
  Sum5/1 -> Mem_Palv/1, BC2/2  "Palv_next"
  Sum7/1 -> Product1/1  "Psw'"
  d_min1/1(bus1) -> deco_stop_time_1/1(bus1)
  d_min2/1(bus1) -> deco_stop_time_2/1(bus1)
  d_min2/2(d_min) -> Mux/2
  In1/1 -> d_min1/2(In1)
  Mem_Palv/1 -> BC1/6  "Palv_next"
  Psw/1 -> Switch2/3
  Switch2/1 -> Mux3/1
  Memory2/1 -> Switch2/1  "Psw_nwxt"
  deco_stop_time_1/1(Pt_new) -> d_min1/1(Pt_new)
  dPsw_next/1 -> Sum/2
  Sum/1 -> BC2/1  "Pstop_next"
  deco_stop_time_2/1(Pt_new) -> d_min2/1(Pt_new)  "Pt_new"
  Sum2/1 -> BC2/3, Sum3/2  "stop_time"
  fcn1/1 -> Sum2/2
  Sum6/1 -> fcn1/1, Switch3/3
  >=0_/1 -> Sum6/2
  Suface/1 -> Relational Operator/2
  Relational Operator/1 -> While Iterator/1
  Sum1/1 -> Mem_ceiling/1
  Mem_ceiling/1 -> ceiling/1, Sum1/2
  Switch1/1 -> Sum1/1
  Mem_ceiling_time/1 -> ceiling_time/1, Sum4/2
  Sum8/1 -> TTS/1
  Palv/1 -> BC1/4  "Palv"
  BC1/1 -> d_min1/3(In2), d_min15/3(In2), d_min16/3(In2), d_min14/3(In2), d_min13/3(In2), d_min12/3(In2), d_min11/3(In2), d_min10/3(In2), d_min9/3(In2), d_min8/3(In2), d_min7/3(In2), d_min6/3(In2), d_min5/3(In2), d_min4/3(In2), d_min3/3(In2), d_min2/3(In2), d_min1b/3(In2)
  In2/1 -> d_min2/2(In1)
  BC2/1 -> deco_stop_time_1/2(bus2), deco_stop_time_15/2(bus2), deco_stop_time_16/2(bus2), deco_stop_time_14/2(bus2), deco_stop_time_13/2(bus2), deco_stop_time_12/2(bus2), deco_stop_time_11/2(" bus2"), deco_stop_time_10/2(bus2), deco_stop_time_9/2(bus2), deco_stop_time_8/2(bus2), deco_stop_time_7/2(bus2), deco_stop_time_6/2(bus2), deco_stop_time_5/2(bus2), deco_stop_time_4/2(bus2), deco_stop_time_3/2(bus2), deco_stop_time_2/2(bus2), deco_stop_time_1b/2(bus2)
  zero/1 -> Switch1/1, Switch3/1
  While Iterator/1 -> BC1/3, Switch2/2, Switch3/2, Switch1/2  "while"
  d_min3/1(bus1) -> deco_stop_time_3/1(bus1)
  deco_stop_time_3/1(Pt_new) -> d_min3/1(Pt_new)
  In3/1 -> d_min3/2(In1)
  In4/1 -> d_min4/2(In1)
  deco_stop_time_4/1(Pt_new) -> d_min4/1(Pt_new)
  d_min4/1(bus1) -> deco_stop_time_4/1(bus1)
  d_min5/1(bus1) -> deco_stop_time_5/1(bus1)
  deco_stop_time_5/1(Pt_new) -> d_min5/1(Pt_new)
  In5/1 -> d_min5/2(In1)
  In6/1 -> d_min6/2(In1)
  deco_stop_time_6/1(Pt_new) -> d_min6/1(Pt_new)
  d_min6/1(bus1) -> deco_stop_time_6/1(bus1)
  d_min7/1(bus1) -> deco_stop_time_7/1(bus1)
  deco_stop_time_7/1(Pt_new) -> d_min7/1(Pt_new)
  In7/1 -> d_min7/2(In1)
  In8/1 -> d_min8/2(In1)
  deco_stop_time_8/1(Pt_new) -> d_min8/1(Pt_new)
  d_min8/1(bus1) -> deco_stop_time_8/1(bus1)
  d_min9/1(bus1) -> deco_stop_time_9/1(bus1)
  deco_stop_time_9/1(Pt_new) -> d_min9/1(Pt_new)
  In9/1 -> d_min9/2(In1)
  In10/1 -> d_min10/2(In1)
  deco_stop_time_10/1(Pt_new) -> d_min10/1(Pt_new)
  d_min10/1(bus1) -> deco_stop_time_10/1(bus1)
  d_min11/1(bus1) -> deco_stop_time_11/1(bus1)
  deco_stop_time_11/1(Pt_new) -> d_min11/1(Pt_new)
  In11/1 -> d_min11/2(In1)
  In12/1 -> d_min12/2(In1)
  deco_stop_time_12/1(Pt_new) -> d_min12/1(Pt_new)
  d_min12/1(bus1) -> deco_stop_time_12/1(bus1)
  d_min13/1(bus1) -> deco_stop_time_13/1(bus1)
  deco_stop_time_13/1(Pt_new) -> d_min13/1(Pt_new)
  In13/1 -> d_min13/2(In1)
  In14/1 -> d_min14/2(In1)
  deco_stop_time_14/1(Pt_new) -> d_min14/1(Pt_new)
  d_min14/1(bus1) -> deco_stop_time_14/1(bus1)
  d_min15/1(bus1) -> deco_stop_time_15/1(bus1)
  deco_stop_time_15/1(Pt_new) -> d_min15/1(Pt_new)
  In15/1 -> d_min15/2(In1)
  In16/1 -> d_min16/2(In1)
  deco_stop_time_16/1(Pt_new) -> d_min16/1(Pt_new)
  d_min16/1(bus1) -> deco_stop_time_16/1(bus1)
  Mux1/1 -> Max1/1
  deco_stop_time_2/2(deco_stop_time) -> Mux1/2
  d_min3/2(d_min) -> Mux/3
  d_min4/2(d_min) -> Mux/4
  d_min5/2(d_min) -> Mux/5
  d_min6/2(d_min) -> Mux/6
  d_min7/2(d_min) -> Mux/7
  d_min8/2(d_min) -> Mux/8
  d_min9/2(d_min) -> Mux/9
  d_min10/2(d_min) -> Mux/10
  d_min11/2(d_min) -> Mux/11
  d_min12/2(d_min) -> Mux/12
  d_min13/2(d_min) -> Mux/13
  d_min14/2(d_min) -> Mux/14
  d_min15/2(d_min) -> Mux/15
  d_min16/2(d_min) -> Mux/16
  deco_stop_time_3/2(deco_stop_time) -> Mux1/3
  deco_stop_time_4/2(deco_stop_time) -> Mux1/4
  deco_stop_time_5/2(deco_stop_time) -> Mux1/5
  deco_stop_time_6/2(deco_stop_time) -> Mux1/6
  deco_stop_time_7/2(deco_stop_time) -> Mux1/7
  deco_stop_time_8/2(deco_stop_time) -> Mux1/8
  deco_stop_time_9/2(deco_stop_time) -> Mux1/9
  deco_stop_time_10/2(deco_stop_time) -> Mux1/10
  deco_stop_time_11/2(deco_stop_time) -> Mux1/11
  deco_stop_time_12/2(deco_stop_time) -> Mux1/12
  deco_stop_time_13/2(deco_stop_time) -> Mux1/13
  deco_stop_time_14/2(deco_stop_time) -> Mux1/14
  deco_stop_time_15/2(deco_stop_time) -> Mux1/15
  deco_stop_time_16/2(deco_stop_time) -> Mux1/16
  Sum4/1 -> Mem_ceiling_time/1
  Switch3/1 -> Sum4/1
  d_min1b/1(bus1) -> deco_stop_time_1b/1(bus1)
  deco_stop_time_1b/1(Pt_new) -> d_min1b/1(Pt_new)
  In1b/1 -> d_min1b/2(In1)
  d_min1b/2(d_min) -> Mux/17
  deco_stop_time_1b/2(deco_stop_time) -> Mux1/17

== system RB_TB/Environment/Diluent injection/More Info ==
  note: Automatic Diluent Valve (ADV) or demand valve or under pressure valve

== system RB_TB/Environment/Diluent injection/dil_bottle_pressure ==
  note: Model: RB_TB/Environment/Diluent injection/pr_dil_bottle
  gas_mix : Inport  Port=1  LatchInput=off
  F_D : Inport  Port=2  LatchInput=off
  Fcn : Fcn  Expr=u(1)/u(2)
  Multiport Switch : MultiPortSwitch  Inputs=2
  Multiport Switch1 : MultiPortSwitch  Inputs=2
  Mux : Mux  Inputs=2
  Product : Product
  Product2 : Product
  Sum : Sum  Inputs=+-
  Sum2 : Sum  Inputs=+-
  Sw1 : MultiPortSwitch  Inputs=3
  Sw4 : MultiPortSwitch  Inputs=3
  integral1 : Integrator
  integral2 : Integrator
  pr_dil_bottle1_ini : Constant  Value=230
  pr_dil_bottle2_ini : Constant  Value=230
  size_dil_bottle1 : Constant  Value=3
  size_dil_bottle2 : Constant  Value=3
  zero : Constant  Value=0
  O2 : Outport
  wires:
  Product/1 -> Sum/1  "vol_dil_bottle1_ini"
  integral1/1 -> Sum/2
  gas_mix/1 -> Sw1/1, Sw4/1, Multiport Switch/1, Multiport Switch1/1
  Sum/1 -> Multiport Switch/2
  Multiport Switch/1 -> Mux/1  "vol_dil_bottle"
  Sw1/1 -> integral1/1
  zero/1 -> Sw4/2, Sw1/3, Sw1/4, Sw4/4
  F_D/1 -> Sw1/2, Sw4/3
  Mux/1 -> Fcn/1
  Fcn/1 -> O2/1  "pr_dil_bottle"
  size_dil_bottle1/1 -> Product/1, Multiport Switch1/2
  pr_dil_bottle1_ini/1 -> Product/2
  Product2/1 -> Sum2/1  "vol_dil_bottle2_ini"
  integral2/1 -> Sum2/2
  Sw4/1 -> integral2/1
  size_dil_bottle2/1 -> Product2/1, Multiport Switch1/3
  pr_dil_bottle2_ini/1 -> Product2/2
  Sum2/1 -> Multiport Switch/3
  Multiport Switch1/1 -> Mux/2  "size_dil_bottle"

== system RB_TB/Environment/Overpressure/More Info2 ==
  note: EN14143:2003(E) 5.6.5 Exhaust valve The exhaust valve shall prevent the pressure in the breathing circuit exceeding 40 mbar. The operation of the exhaust valve shall not be degraded after being subjected to a) a constant flow of 300 l min-1 for a period of 1 min; 6.5 Breathable volume 6.5.1 Volume The internal pressure when withdrawing the gas shall not exceed - 25 mbar and when injecting gas + 25 mbar.

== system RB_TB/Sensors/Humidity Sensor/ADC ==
  note: Model: RB_TB/Sensors/Humidity_sensor/ADC
  note: This subsystem models a typical 16-bit analog-to-digital converter having an input range of 0-5 volts
  voltage : Inport  Port=1  LatchInput=off
  limit : Saturate  UpperLimit=65535  LowerLimit=0
  quantize : Quantizer  QuantizationInterval=1
  scale : Gain  Gain=65536/5
  pcm : Outport
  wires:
  limit/1 -> pcm/1
  scale/1 -> quantize/1
  quantize/1 -> limit/1
  voltage/1 -> scale/1

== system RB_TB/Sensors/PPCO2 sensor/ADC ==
  note: This subsystem models a typical 16-bit analog-to-digital converter having an input range of 0-5 volts
  note: Model: RB_TB/Sensors/PPCO2 sensor/ADC
  voltage : Inport  Port=1  LatchInput=off
  limit : Saturate  UpperLimit=65535  LowerLimit=0
  quantize : Quantizer  QuantizationInterval=1
  scale : Gain  Gain=65536/5
  pcm : Outport
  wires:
  voltage/1 -> scale/1
  quantize/1 -> limit/1
  scale/1 -> quantize/1
  limit/1 -> pcm/1

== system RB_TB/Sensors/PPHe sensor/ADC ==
  note: Model: RB_TB/Sensors/PPO2 sensor/ADC
  note: This subsystem models a typical 16-bit analog-to-digital converter having an input range of 0-5 volts
  voltage : Inport  Port=1  LatchInput=off
  limit : Saturate  UpperLimit=65535  LowerLimit=0
  quantize : Quantizer  QuantizationInterval=1
  scale : Gain  Gain=65536/5
  pcm : Outport
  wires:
  voltage/1 -> scale/1
  quantize/1 -> limit/1
  scale/1 -> quantize/1
  limit/1 -> pcm/1

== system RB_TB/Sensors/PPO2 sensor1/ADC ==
  note: Model: RB_TB/Sensors/PPO2 sensor/ADC
  note: This subsystem models a typical 16-bit analog-to-digital converter having an input range of 0-5 volts
  voltage : Inport  Port=1  LatchInput=off
  limit : Saturate  UpperLimit=65535  LowerLimit=0
  quantize : Quantizer  QuantizationInterval=1
  scale : Gain  Gain=65536/5
  pcm : Outport
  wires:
  voltage/1 -> scale/1
  quantize/1 -> limit/1
  scale/1 -> quantize/1
  limit/1 -> pcm/1

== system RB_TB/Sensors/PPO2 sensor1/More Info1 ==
  note: Sensor fusion by using a sliding observer for an underwater breathing system Salvatore Carotenuto, Luigi Iannelli, Sabato Manfredi, Stefania Santini e-mail: luigi.iannelli@unisannio.it, {salcarot, smanfred, stsantin}@unina.it ... When working in critical conditions or environments, such as under the sea, the control-loop has to be fault-tolerant. In other words the control strategy of the rebreather system has to be 'robust' against sensor failures. An error on the actual oxygen level measurement, especially in the set point proximity, can cause a disease to the diver and may have fatal consequences. Thus, in the counterlung control-loop some hardware redundancy is desired: usually the system output (oxygen partial pressure) is measured through three sensors so that eventual sensor faults can be detected and isolated for the diver safety. Of course, by introducing this redundancy, an algorithm that decides which measurement value to give to the controller is needed. The problem of designing this algorithm is called 'sensor fusion' problem. ... The performance of the proposed strategy are discussed comparing it with a more traditional approach based on a decision by majority criteria [7], [8], usually named as voting logic, which is currently implemented in some commercial rebreathers and is a proven technology in some applicative areas as fly-by-wire control [9].
  note: Terminology:

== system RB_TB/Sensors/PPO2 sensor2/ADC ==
  note: This subsystem models a typical 16-bit analog-to-digital converter having an input range of 0-5 volts
  note: Model: RB_TB/Sensors/PPO2 sensor/ADC
  voltage : Inport  Port=1  LatchInput=off
  limit : Saturate  UpperLimit=65535  LowerLimit=0
  quantize : Quantizer  QuantizationInterval=1
  scale : Gain  Gain=65536/5
  pcm : Outport
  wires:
  limit/1 -> pcm/1
  scale/1 -> quantize/1
  quantize/1 -> limit/1
  voltage/1 -> scale/1

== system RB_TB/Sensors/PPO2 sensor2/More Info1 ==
  note: Terminology:
  note: Sensor fusion by using a sliding observer for an underwater breathing system Salvatore Carotenuto, Luigi Iannelli, Sabato Manfredi, Stefania Santini e-mail: luigi.iannelli@unisannio.it, {salcarot, smanfred, stsantin}@unina.it ... When working in critical conditions or environments, such as under the sea, the control-loop has to be fault-tolerant. In other words the control strategy of the rebreather system has to be 'robust' against sensor failures. An error on the actual oxygen level measurement, especially in the set point proximity, can cause a disease to the diver and may have fatal consequences. Thus, in the counterlung control-loop some hardware redundancy is desired: usually the system output (oxygen partial pressure) is measured through three sensors so that eventual sensor faults can be detected and isolated for the diver safety. Of course, by introducing this redundancy, an algorithm that decides which measurement value to give to the controller is needed. The problem of designing this algorithm is called 'sensor fusion' problem. ... The performance of the proposed strategy are discussed comparing it with a more traditional approach based on a decision by majority criteria [7], [8], usually named as voting logic, which is currently implemented in some commercial rebreathers and is a proven technology in some applicative areas as fly-by-wire control [9].

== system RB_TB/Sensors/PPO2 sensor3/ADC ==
  note: Model: RB_TB/Sensors/PPO2 sensor/ADC
  note: This subsystem models a typical 16-bit analog-to-digital converter having an input range of 0-5 volts
  voltage : Inport  Port=1  LatchInput=off
  limit : Saturate  UpperLimit=65535  LowerLimit=0
  quantize : Quantizer  QuantizationInterval=1
  scale : Gain  Gain=65536/5
  pcm : Outport
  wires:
  voltage/1 -> scale/1
  quantize/1 -> limit/1
  scale/1 -> quantize/1
  limit/1 -> pcm/1

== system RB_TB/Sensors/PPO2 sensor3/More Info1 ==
  note: Sensor fusion by using a sliding observer for an underwater breathing system Salvatore Carotenuto, Luigi Iannelli, Sabato Manfredi, Stefania Santini e-mail: luigi.iannelli@unisannio.it, {salcarot, smanfred, stsantin}@unina.it ... When working in critical conditions or environments, such as under the sea, the control-loop has to be fault-tolerant. In other words the control strategy of the rebreather system has to be 'robust' against sensor failures. An error on the actual oxygen level measurement, especially in the set point proximity, can cause a disease to the diver and may have fatal consequences. Thus, in the counterlung control-loop some hardware redundancy is desired: usually the system output (oxygen partial pressure) is measured through three sensors so that eventual sensor faults can be detected and isolated for the diver safety. Of course, by introducing this redundancy, an algorithm that decides which measurement value to give to the controller is needed. The problem of designing this algorithm is called 'sensor fusion' problem. ... The performance of the proposed strategy are discussed comparing it with a more traditional approach based on a decision by majority criteria [7], [8], usually named as voting logic, which is currently implemented in some commercial rebreathers and is a proven technology in some applicative areas as fly-by-wire control [9].
  note: Terminology:

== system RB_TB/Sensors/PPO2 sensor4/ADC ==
  note: This subsystem models a typical 16-bit analog-to-digital converter having an input range of 0-5 volts
  note: Model: RB_TB/Sensors/PPO2 sensor/ADC
  voltage : Inport  Port=1  LatchInput=off
  limit : Saturate  UpperLimit=65535  LowerLimit=0
  quantize : Quantizer  QuantizationInterval=1
  scale : Gain  Gain=65536/5
  pcm : Outport
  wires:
  limit/1 -> pcm/1
  scale/1 -> quantize/1
  quantize/1 -> limit/1
  voltage/1 -> scale/1
